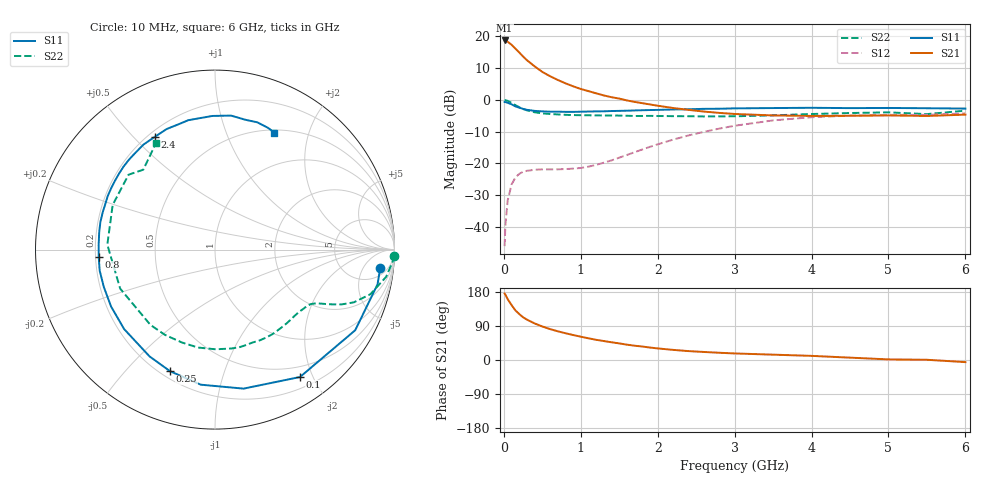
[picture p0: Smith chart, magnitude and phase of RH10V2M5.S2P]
! SIEMENS Small Signal Semiconductors
! BFR106
! Si NPN RF Bipolar Junction Transistor in SOT23
! VCE = 10 V  IC = 2.5 mA
! Common Emitter S-Parameters:  August  1996
# GHz  S  MA  R  50
!  f  S11  S21  S12  S22
! GHz  MAG  ANG  MAG  ANG  MAG  ANG  MAG  ANG
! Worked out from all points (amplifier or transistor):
!   36 points, 10 MHz to 6 GHz, reference 50 ohm
!   highest |S21| = 18.7 dB at 10 MHz (marker M1)
!   |S21| within 3 dB of that: start of sweep to 168.2 MHz
!   unconditionally stable (mu >= 1): 755.5 MHz to 1.82 GHz; 4.346 GHz to end of sweep
!   at 250 MHz: K = 0.35, MSG = 18.1 dB, |S12| = -22.6 dB
!   at 1.4 GHz: K = 1.21, MAG = 7.2 dB, |S12| = -19.0 dB
!   at 6 GHz: K = 1.02, MAG = -1.1 dB, |S12| = -4.2 dB
!   S11 on the Smith chart (normalised r, x): 10 MHz: 9, -12; 100 MHz: 0.35, -1.82; 250 MHz: 0.24, -0.67; 800 MHz: 0.21, -0.03; 2.4 GHz: 0.23, +0.58; 6 GHz: 0.53, +1.49
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0.01  0.9266 -6.2  8.62 175.4  0.005 89.4  0.9975 -1.9
0.02  0.926 -12.1  8.597 172.3  0.0105 85.5  0.9925 -3.8
0.05  0.9012 -29.9  8.23 160.6  0.0262 73.3  0.9659 -9.0
0.1  0.8533 -56.3  7.386 145.1  0.0466 61.2  0.9011 -16.0
0.15  0.7907 -78.4  6.424 130.9  0.0601 50.5  0.8275 -20.8
0.2  0.7568 -96.0  5.58 121.3  0.0686 43.9  0.7688 -23.4
0.25  0.7223 -110.3  4.82 112.7  0.0742 38.7  0.7191 -25.1
0.3  0.6979 -121.5  4.219 106.6  0.0767 35.9  0.6862 -26.2
0.4  0.6726 -138.8  3.374 96.5  0.0796 32.1  0.6388 -27.9
0.5  0.6602 -151.3  2.76 88.4  0.0808 31.1  0.6143 -29.6
0.6  0.6535 -161.4  2.363 81.6  0.0809 32.2  0.6005 -31.7
0.8  0.6492 -176.2  1.828 70.7  0.0816 37.6  0.5826 -36.7
1.1  0.6569 166.4  1.375 57.3  0.0891 52.0  0.5728 -45.9
1.6  0.6769 145.2  0.981 40.5  0.1361 69.6  0.5638 -63.8
2.2  0.7078 124.3  0.746 26.7  0.2372 70.5  0.5555 -89.6
2.4  0.7126 117.9  0.698 23.5  0.2759 68.0  0.5538 -99.8
3  0.7361 101.7  0.601 17.3  0.3921 56.3  0.5526 -130.7
3.5  0.7447 91.2  0.57 14.1  0.4762 44.5  0.5713 -157.6
4.5  0.7429 76.8  0.563 6.2  0.5659 21.8  0.6221 156.4
5  0.7474 71.6  0.57 1.6  0.5821 12.8  0.6372 139.1
5.5  0.7396 66.3  0.559 0.6  0.5823 8.3  0.5982 131.9
6  0.7307 63.1  0.587 -5.6  0.6144 -0.1  0.6774 119.1
